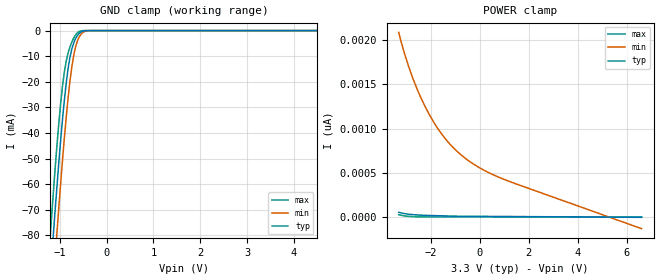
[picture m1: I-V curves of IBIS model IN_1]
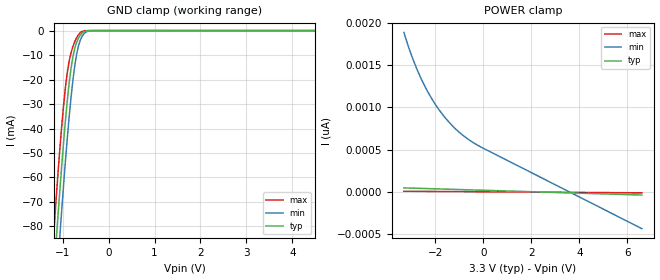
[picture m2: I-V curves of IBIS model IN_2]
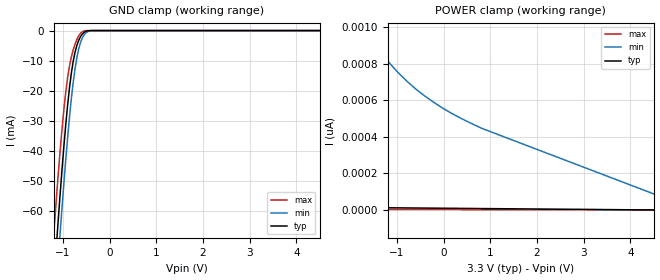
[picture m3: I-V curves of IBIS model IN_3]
|//////////////////////////////////////////////////////////////////////////////
|//////////////////////////////////////////////////////////////////////////////
|   @@@@@@@   @@@@@@@   @@@@@@@   @@@@@@@   @@@@@@@   @@@@@@   @@
|   @@@@@@@@@   @@@@@@@@@   @@@@@@@@@   @@@@@@@@@   @@@@@@@@@ @@@@@@@@  @
|   @@@   @@@ @@@   @@@ @@@   @@@   @@@ @@@   @@@@   @@@  @
|   @@   @@ @@   @@ @@@@@@@@@@@ @@@@@@@@@@@ @@   @@   @@ @@
|   @@@   @@@ @@   @@   @@@ @@@   @@   @@   @@ @@
|   @@@@@@@@@  @@   @@  @@@@@@@@@   @@@@@@@@@  @@   @@   @@ @@
|   @@@@@@@   @@   @@   @@@@@@@   @@@@@@@   @@   @@   @@ @@
|   IBIS Model of CAT9532
|   I/O Port Expander, I2C / SMBus, 16-Bit, with LED Dimming
|   Case  948AR, TSSOP-24 Package Type
|   510AG,  TQFN-24 Package Type
|   The device is powered at Vcc = 3.3V.
|//////////////////////////////////////////////////////////////////////////////
|//////////////////////////////////////////////////////////////////////////////
[IBIS Ver]   3.2
|   7.2 compatible
|//////////////////////////////////////////////////////////////////////////////
[Comment Char]  |_char
|//////////////////////////////////////////////////////////////////////////////
[File Name]   cat9532_va_r0.ibs
|//////////////////////////////////////////////////////////////////////////////
[File Rev]   0.0
|   0.0 - Dec 18, 2024 - File created
|//////////////////////////////////////////////////////////////////////////////
[Date]   Dec 18, 2024
|//////////////////////////////////////////////////////////////////////////////
[Notes]
   - The currents greater than +/- 100 mA are extrapolated
|//////////////////////////////////////////////////////////////////////////////
[Disclaimer]
   - onsemi Corporation hereby grants
   the user of this IBIS model a license to use this IBIS
   model under the following terms. This license in nonexclusive
   and nontransferable. Before using this IBIS model.
   After reading the terms and conditions of this license,
   the user either must accept these terms,
   or the IBIS model should be returned to onsemi within 30 days.
   - The user is hereby granted a license to use the IBIS model.
   This shall not be construed as a right to sell,
   or otherwise profit either by leasing or renting this software.
   - The user may modify the IBIS model to suit his specific
   applications but rights to derivative works and such
   modifications shall belong to onsemi.
   - This IBIS model is provided on an "as is" basis.
   onsemi makes absolutely no warranty with respect
   to the information contained herein.
   By use of this IBIS model, the user assumes full risk as to the
   quality and suitablility of the model to his particular use,
   and by using this model assumes the entire risk.
   Under all circumstances the user shall not hold
   onsemi liable in any way for the results obtained.
   onsemi reserves the right to make to improve
   the model for reliability, function, or design.
   onsemi does not convey any license under patent
   rights or any other intellectual property rights,
   including those of third parties.
   - onsemi is not obligated to provide maintenance
   or support for the licensed IBIS model.
   - Cont onsemi at ATTN:LOGIC APPLICATIONS/IBIS MODEL.
   5701 N Pima Rd, Scottsdale, AZ 85250
|//////////////////////////////////////////////////////////////////////////////
[Copyright]   (c) 2024 onsemi Corp.
|//////////////////////////////////////////////////////////////////////////////
|//////////////////////////////////////////////////////////////////////////////
[Component]   CAT9532HV6I-GT2
|//////////////////////////////////////////////////////////////////////////////
[Manufacturer]  onsemi Corp.
|   Data Sheet: CAT9532/D   rev. 6   Nov,2024
|//////////////////////////////////////////////////////////////////////////////
[Package]
| TSSOP-24
| variable   typ   min   max
R_pkg   0.0423   0.0358   0.4397
L_pkg   2.6923nH   2.3682nH   3.1791nH
C_pkg   0.3231pF   0.2587pF   0.4397pF
|//////////////////////////////////////////////////////////////////////////////
[Pin] signal_name   model_name   R_pin   L_pin   C_pin
1   A0   IN_3   0.0371   3.1555nH  0.4397pF
2   A1   IN_3   0.0367   2.6293nH  0.3427pF
3   A2   IN_3   0.0367   2.8663nH  0.3477pF
4   LED0   I/O_2   0.0446   2.7479nH  0.2993pF
5   LED1   I/O_2   0.0482   2.6830nH  0.2631pF
6   LED2   I/O_2   0.0486   2.4181nH  0.2695pF
7   LED3   I/O_2   0.0493   2.3682nH  0.2659pF
8   LED4   I/O_2   0.0487   2.4698nH  0.2590pF
9   LED5   I/O_2   0.0488   2.5485nH  0.2764pF
10   LED6   I/O_2   0.0358   2.6199nH  0.3322pF
11   LED7   I/O_2   0.0387   2.6799nH  0.3466pF
12   VSS   GND   0.0399   3.1791nH  0.4370pF
13   LED8   I/O_2   0.0372   3.1140nH  0.4395pF
14   LED9   I/O_2   0.0374   2.6565nH  0.3463pF
15   LED10   I/O_2   0.0366   2.7396nH  0.3445pF
16   LED11   I/O_2   0.0463   2.6494nH  0.2826pF
17   LED12   I/O_2   0.0473   2.5358nH  0.2595pF
18   LED13   I/O_2   0.0441   2.4292nH  0.2677pF
19   LED14   I/O_2   0.0460   2.4267nH  0.2662pF
20   LED15   I/O_2   0.0465   2.5353nH  0.2587pF
21   RESET   IN_2   0.0478   2.6488nH  0.2859pF
22   SCL   IN_1   0.0369   2.7389nH  0.3398pF
23   SDA   I/O_1   0.0386   2.6564nH  0.3448pF
24   VCC   POWER   0.0384   3.1188nH  0.4391pF
|//////////////////////////////////////////////////////////////////////////////
|//////////////////////////////////////////////////////////////////////////////
[Component]   CAT9532YI-T2
|//////////////////////////////////////////////////////////////////////////////
[Manufacturer]  onsemi Corp.
|   Data Sheet: CAT9532/D   rev. 6   Nov,2024
|//////////////////////////////////////////////////////////////////////////////
[Package]
| TQFN-24
| variable   typ   min   max
R_pkg   0.0386   0.0238   0.3209
L_pkg   0.6535nH   0.1332nH   0.9554nH
C_pkg   0.2561pF   0.2316pF   0.3209pF
|//////////////////////////////////////////////////////////////////////////////
[Pin] signal_name   model_name   R_pin   L_pin   C_pin
1   LED0   I/O_2   0.0348   0.7269nH  0.2479pF
2   LED1   I/O_2   0.0357   0.6233nH  0.2688pF
3   LED2   I/O_2   0.0376   0.6360nH  0.2703pF
4   LED3   I/O_2   0.0314   0.6168nH  0.2689pF
5   LED4   I/O_2   0.0319   0.6723nH  0.2685pF
6   LED5   I/O_2   0.0310   0.7963nH  0.2617pF
7   LED6   I/O_2   0.0351   0.7311nH  0.2677pF
8   LED7   I/O_2   0.0396   0.9554nH  0.2648pF
9   VSS   GND   0.0474   0.9294nH  0.2597pF
10   LED8   I/O_2   0.0492   0.8350nH  0.2316pF
11   LED9   I/O_2   0.0443   0.1484nH  0.2557pF
12   LED10   I/O_2   0.0389   0.7664nH  0.2405pF
13   LED11   I/O_2   0.0339   0.7459nH  0.2604pF
14   LED12   I/O_2   0.0395   0.7584nH  0.2373pF
15   LED13   I/O_2   0.0238   0.6998nH  0.2405pF
16   LED14   I/O_2   0.0371   0.6673nH  0.2338pF
17   LED15   I/O_2   0.0329   0.7223nH  0.2321pF
18   RESET   IN_2   0.0346   0.8691nH  0.2541pF
19   SCL   IN_1   0.0398   0.7329nH  0.2326pF
20   SDA   I/O_1   0.0453   0.1361nH  0.2593pF
21   VCC   POWER   0.0467   0.8467nH  0.2361pF
22   A0   IN_3   0.0471   0.1332nH  0.3209pF
23   A1   IN_3   0.0577   0.1598nH  0.2833pF
24   A2   IN_3   0.0311   0.7756nH  0.2492pF
| Models and submodels in the file (5): IN_1 (Input), IN_2 (Input), IN_3 (Input), I/O_1 (I/O_open_drain), I/O_2 (I/O_open_drain)
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|//////////////////////////////////////////////////////////////////////////////
|//////////////////////////////////////////////////////////////////////////////
[Model]  IN_1
Model_type Input
Vinh = 2.31
Vinl = 0.99
|  variable   typ   min   max
C_comp   3.022pF   3.022pF   3.022pF
|//////////////////////////////////////////////////////////////////////////////
[Temperature Range]   25   85   -40
|//////////////////////////////////////////////////////////////////////////////
[Voltage Range]   3.30V   3.0V   3.60V
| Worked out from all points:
|   GND clamp passes 1 mA (typ) near -0.58 V on its own axis
|//////////////////////////////////////////////////////////////////////////////
[GND Clamp]
|   Voltage   I(typ)   I(min)  I(max)
-3.3V     -645.8mA   -642.1mA   -651.1mA
-1.22V    -101.9mA   -120.1mA   -85.43mA
-1.18V    -91.4mA    -110mA     -74.86mA
-1.14V    -81.13mA   -99.98mA   -64.59mA
-1.1V     -71.1mA    -89.77mA   -54.73mA
-1.06V    -61.45mA   -79.64mA   -45.42mA
-940mV    -34.84mA   -50.86mA   -21.84mA
-820mV    -14.86mA   -26.37mA   -8.759mA
-700mV    -4.808mA   -9.684mA   -2.886mA
-580mV    -1.043mA   -2.4mA     -322.1uA
-340mV    -772.5nA   -11.92uA   -10.95nA
6.6V      12.63pA    906.1pA    245.9fA
|//////////////////////////////////////////////////////////////////////////////
[POWER Clamp]
|   Voltage   I(typ)   I(min)  I(max)
-3.3V     53.6pA     2.089nA    25.37pA
-3.04V    36.88pA    1.831nA    11.09pA
-2.76V    27.08pA    1.598nA    4.051pA
-2.48V    21.75pA    1.403nA    1.379pA
-2.16V    17.82pA    1.216nA    385.1fA
-1.84V    15.17pA    1.059nA    200.8fA
-1.48V    12.42pA    914pA      186.8fA
-1.12V    9.849pA    797.7pA    172.9fA
-680mV    8.193pA    684.9pA    155.8fA
40mV      6.971pA    550.1pA    127.8fA
960mV     5.413pA    429pA      92.06fA
6.6V      -4.137pA   -132.5pA   -127fA
|//////////////////////////////////////////////////////////////////////////////
|//////////////////////////////////////////////////////////////////////////////
[Model]  IN_2
Model_type Input
Vinh = 2.31
Vinl = 0.66
|  variable   typ   min   max
C_comp   3pF   3pF   3pF
|//////////////////////////////////////////////////////////////////////////////
[Temperature Range]   25   85   -40
|//////////////////////////////////////////////////////////////////////////////
[Voltage Range]   3.30V   3.0V   3.60V
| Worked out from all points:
|   GND clamp passes 1 mA (typ) near -0.58 V on its own axis
|//////////////////////////////////////////////////////////////////////////////
[GND Clamp]
|   Voltage   I(typ)   I(min)   I(max)
-3.3V     -680.4mA   -681.5mA   -681.3mA
-1.22V    -107.5mA   -126mA     -89.78mA
-1.18V    -96.45mA   -115.3mA   -78.67mA
-1.14V    -85.53mA   -104.6mA   -67.9mA
-1.1V     -74.9mA    -93.96mA   -57.58mA
-1.06V    -64.69mA   -83.29mA   -47.82mA
-940mV    -36.62mA   -53.13mA   -23.07mA
-820mV    -15.54mA   -27.53mA   -9.132mA
-700mV    -4.936mA   -9.986mA   -3.004mA
-580mV    -1.05mA    -2.388mA   -349.7uA
-340mV    -4.321uA   -14.04uA   -4.937uA
6.6V      47.96pA    1.121nA    7.559pA
|//////////////////////////////////////////////////////////////////////////////
[POWER Clamp]
|   Voltage   I(typ)   I(min)  I(max)
-3.3V     47.96pA    1.889nA    8.13pA
-3.08V    46.08pA    1.694nA    7.711pA
-2.84V    44.02pA    1.51nA     7.255pA
-2.56V    41.63pA    1.327nA    6.722pA
-2.28V    39.23pA    1.172nA    6.19pA
-1.96V    36.49pA    1.023nA    5.581pA
-1.64V    33.75pA    898.8pA    4.973pA
-1.28V    30.67pA    782.2pA    4.288pA
-920mV    27.59pA    687.9pA    3.604pA
-520mV    24.16pA    603.4pA    2.843pA
-80mV     20.39pA    529.2pA    2.006pA
6.6V      -36.8pA    -434.8pA   -10.7pA
|//////////////////////////////////////////////////////////////////////////////
|//////////////////////////////////////////////////////////////////////////////
[Model]  IN_3
Model_type Input
Vinh = 2.0
Vinl = 0.8
|  variable   typ   min   max
C_comp   3.4pF   3.4pF   3.4pF
|//////////////////////////////////////////////////////////////////////////////
[Temperature Range]   25   85   -40
|//////////////////////////////////////////////////////////////////////////////
[Voltage Range]   3.30V   3.0V   3.60V
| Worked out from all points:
|   GND clamp passes 1 mA (typ) near -0.57 V on its own axis
|//////////////////////////////////////////////////////////////////////////////
[GND Clamp]
|   Voltage   I(typ)   I(min)  I(max)
-3.3V     -575.5mA   -576.4mA   -569.8mA
-1.22V    -90.32mA   -103.5mA   -73.44mA
-1.18V    -81.13mA   -94.39mA   -64.7mA
-1.14V    -72.11mA   -85.34mA   -56.21mA
-1.1V     -63.34mA   -76.47mA   -48.07mA
-1.06V    -54.87mA   -67.87mA   -40.4mA
-940mV    -31.73mA   -43.45mA   -20.82mA
-820mV    -14.38mA   -22.95mA   -8.914mA
-700mV    -4.946mA   -8.988mA   -2.986mA
-580mV    -1.084mA   -2.353mA   -345.2uA
-340mV    -813.5nA   -11.94uA   -12.71nA
6.6V      15.22pA    877.3pA    1.902pA
|//////////////////////////////////////////////////////////////////////////////
[POWER Clamp]
|   Voltage   I(typ)   I(min)  I(max)
-3.3V     127.2pA    4.22nA     1.99pA
-3.12V    70.62pA    2.9nA      1.937pA
-3V       50.59pA    2.392nA    1.902pA
-2.84V    35.82pA    2.007nA    1.854pA
-1.68V    13.88pA    986.4pA    1.512pA
-1.48V    12.28pA    908.9pA    1.453pA
-1.24V    10.83pA    828.8pA    1.383pA
-760mV    9.81pA     698.7pA    1.241pA
-240mV    8.703pA    594.2pA    1.088pA
380mV     7.384pA    500pA      904.9fA
820mV     6.447pA    446pA      775.1fA
6.6V      -5.857pA   -118.1pA   -929.3fA
